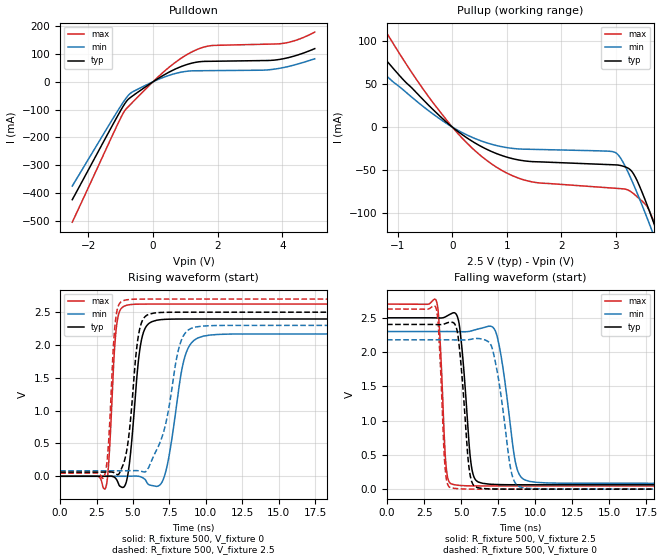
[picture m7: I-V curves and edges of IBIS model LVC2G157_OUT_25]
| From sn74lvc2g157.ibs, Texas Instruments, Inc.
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[Model]   LVC2G157_OUT_25
Model_type  Output
Vref =   0
Rref =   500
Cref =   30p
Vmeas =   1.25
| variable   typ   min   max
C_comp   9.71pF   6.17pF   14.70pF
| C_pullup   9.39pF   6.17pF   11.05pF
| C_pulldown   10.02pF   6.58pF   14.70pF
[Temperature Range]   40   100   -40
| Ambient temperature   25   85   -40
[Voltage range]   2.5   2.3   2.7
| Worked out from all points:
|   slope of the pulldown table from 0 to 0.375 V, typ, clamps not added: 13.9 ohm
|   slope of the pullup table from 0 to 0.375 V, typ, clamps not added: 22.2 ohm
|   rising waveform, R_fixture 500, V_fixture 0: 20-80 % time 571ps typ, 888ps min, 367ps max; typ from 0 V to 2.4 V
|   falling waveform, R_fixture 500, V_fixture 2.5: 20-80 % time 506ps typ, 796ps min, 326ps max; typ from 2.5 V to 0.063 V
|   rising waveform, R_fixture 500, V_fixture 2.5: 20-80 % time 611ps typ, 1.18ns min, 373ps max; typ from 0.063 V to 2.5 V
|   falling waveform, R_fixture 500, V_fixture 0: 20-80 % time 506ps typ, 828ps min, 320ps max; typ from 2.4 V to 0 V
[Pulldown]
| LVC2G157_OUT_25
|   Voltage   I(typ)   I(min)   I(max)
-2.5V     -423.8mA   -374.7mA   -504.6mA
-900mV    -83.31mA   -69.6mA    -107.9mA
-780mV    -64.42mA   -50.73mA   -91.1mA
-625mV    -50.16mA   -35.79mA   -72.59mA
125mV     9.48mA     6.528mA    14.01mA
590mV     40.15mA    26.41mA    60.88mA
1.15V     65.36mA    38.83mA    104.2mA
1.65V     73.22mA    39.77mA    126.8mA
3.41V     76.05mA    41.66mA    134.7mA
3.995V    81.88mA    50.05mA    137.4mA
4.47V     95.98mA    63.45mA    151mA
5V        118.9mA    82.47mA    178.4mA
[Pullup]
| LVC2G157_OUT_25
|   Voltage   I(typ)   I(min)   I(max)
-2.5V     184.4mA    145.2mA    258.3mA
-2.065V   146.4mA    114.6mA    205.8mA
-1.655V   112.2mA    87.22mA    158.5mA
-1.285V   83.12mA    64.1mA     117.9mA
45mV      -2.273mA   -1.669mA   -3.327mA
1.03V     -35.39mA   -24.09mA   -54.31mA
1.545V    -40.27mA   -25.93mA   -64.48mA
2.975V    -43.81mA   -28.98mA   -70.99mA
3.32V     -53.5mA    -65.41mA   -76.9mA
3.655V    -103.6mA   -118.3mA   -102.4mA
3.785V    -126.3mA   -140mA     -125.3mA
5V        -356.5mA   -355.8mA   -379.1mA
[Ramp]
| LVC2G157_OUT_25
| variable   typ   min   max
dV/dt_r   1.54/6.12E-10   1.39/9.52E-10   1.69/3.94E-10
dV/dt_f   1.51/5.29E-10   1.38/8.32E-10   1.64/3.42E-10
R_load = 500
[Rising Waveform]
| LVC2G157_OUT_25
R_fixture =   500
C_fixture =   0
L_fixture =   0
V_fixture =   0
V_fixture_min = 0
V_fixture_max = 0
|   Time   V(typ)   V(min)   V(max)
0s        129pV      6.207nV    595.7pV
3.125ns   537.2uV    -27.68uV   -175.7mV
3.84ns    -38.89mV   -13.02uV   2.229V
4.44ns    -145.4mV   250.6uV    2.596V
5.51ns    1.99V      -6.047mV   2.623V
6.295ns   2.355V     -140.7mV   2.624V
7.165ns   2.391V     5.052mV    2.624V
8.475ns   2.396V     1.75V      2.624V
9.485ns   2.396V     2.11V      2.624V
29.99ns   2.396V     2.17V      2.624V
[Falling Waveform]
| LVC2G157_OUT_25
R_fixture =   500
C_fixture =   0
L_fixture =   0
V_fixture =   2.5
V_fixture_min = 2.3
V_fixture_max = 2.7
|   Time   V(typ)   V(min)   V(max)
0s        2.5V       2.3V       2.7V
3.335ns   2.498V     2.3V       2.742V
3.965ns   2.517V     2.3V       378.4mV
4.365ns   2.564V     2.3V       74.94mV
4.86ns    2.418V     2.298V     55.64mV
5.65ns    401.2mV    2.307V     48.35mV
6.18ns    102.1mV    2.339V     47.33mV
7.375ns   68.09mV    2.269V     46.86mV
9.315ns   63.81mV    133.2mV    46.81mV
29.99ns   63.48mV    83.95mV    46.77mV
[Rising Waveform]
| LVC2G157_OUT_25
R_fixture =   500
C_fixture =   0
L_fixture =   0
V_fixture =   2.5
V_fixture_min = 2.3
V_fixture_max = 2.7
|   Time   V(typ)   V(min)   V(max)
0s        63.44mV    83.88mV    46.75mV
3.075ns   63.78mV    83.86mV    34.36mV
3.315ns   65.27mV    83.84mV    485.5mV
3.775ns   45.42mV    83.88mV    2.324V
4.285ns   155.5mV    83.95mV    2.672V
5.385ns   2.16V      83.66mV    2.699V
6.075ns   2.467V     133.4mV    2.7V
8.22ns    2.5V       2.007V     2.7V
9.015ns   2.5V       2.256V     2.7V
29.99ns   2.5V       2.3V       2.7V
[Falling Waveform]
| LVC2G157_OUT_25
R_fixture =   500
C_fixture =   0
L_fixture =   0
V_fixture =   0
V_fixture_min = 0
V_fixture_max = 0
|   Time   V(typ)   V(min)   V(max)
0s        2.403V     2.179V     2.628V
3.29ns    2.402V     2.179V     2.65V
3.91ns    2.413V     2.179V     332.7mV
4.275ns   2.436V     2.179V     22.26mV
4.765ns   2.272V     2.177V     6.993mV
5.52ns    331mV      2.181V     1.247mV
6.005ns   29.6mV     2.198V     482.2uV
7.095ns   3.201mV    2.055V     105.1uV
8.935ns   246.9uV    36.19mV    55.34uV
29.99ns   33.91uV    56.47uV    21.27uV
